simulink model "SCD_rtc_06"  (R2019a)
settings: Solver=VariableStepAuto  StartTime=0.0  StopTime=10.0  RelTol=1e-3
undefined symbols (not defined in the file or in its folder): algo_cfs1_fp

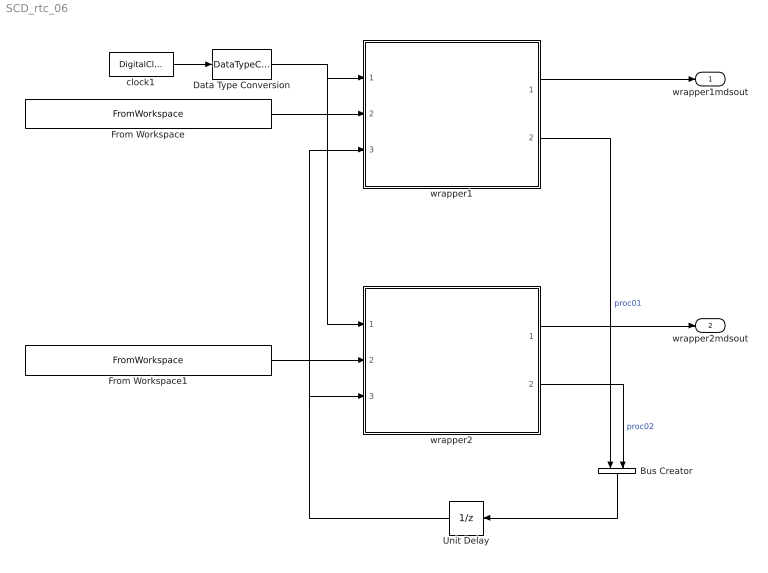
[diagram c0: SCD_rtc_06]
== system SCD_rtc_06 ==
  Bus Creator : BusCreator  Inputs=2
  Data Type Conversion : DataTypeConversion  OutDataTypeStr=single
  From Workspace : FromWorkspace  VariableName=SCDsimdata.SCDnode0601_simdata.wavegen  OutDataTypeStr=Bus: WG0601bus  Interpolate=off  OutputAfterFinalValue=Holding final value
  From Workspace1 : FromWorkspace  VariableName=SCDsimdata.SCDnode0602_simdata.wavegen  OutDataTypeStr=Bus: WG0602bus  Interpolate=off  OutputAfterFinalValue=Holding final value
  Unit Delay : UnitDelay  SampleTime=-1  HasFrameUpgradeWarning=on
  clock1 : DigitalClock  SampleTime=algo_cfs1_fp.timing.dt
  wrapper1 : ModelReference  ModelNameDialog=wrapper1.slx  SimulationMode=Normal  ModelReferenceVersion=1.14
  wrapper2 : ModelReference  ModelNameDialog=wrapper2.slx  SimulationMode=Normal  ModelReferenceVersion=1.7
  wrapper1mdsout : Outport  OutDataTypeStr=Bus: mdsout01
  wrapper2mdsout : Outport  Port=2  OutDataTypeStr=Bus: mdsout02
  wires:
  wrapper1/1 -> wrapper1mdsout/1
  wrapper2/1 -> wrapper2mdsout/1
  wrapper1/2 -> Bus Creator/1  "proc01"
  wrapper2/2 -> Bus Creator/2  "proc02"
  Bus Creator/1 -> Unit Delay/1
  Unit Delay/1 -> wrapper2/3, wrapper1/3
  From Workspace/1 -> wrapper1/2
  clock1/1 -> Data Type Conversion/1
  Data Type Conversion/1 -> wrapper2/1, wrapper1/1
  From Workspace1/1 -> wrapper2/2
